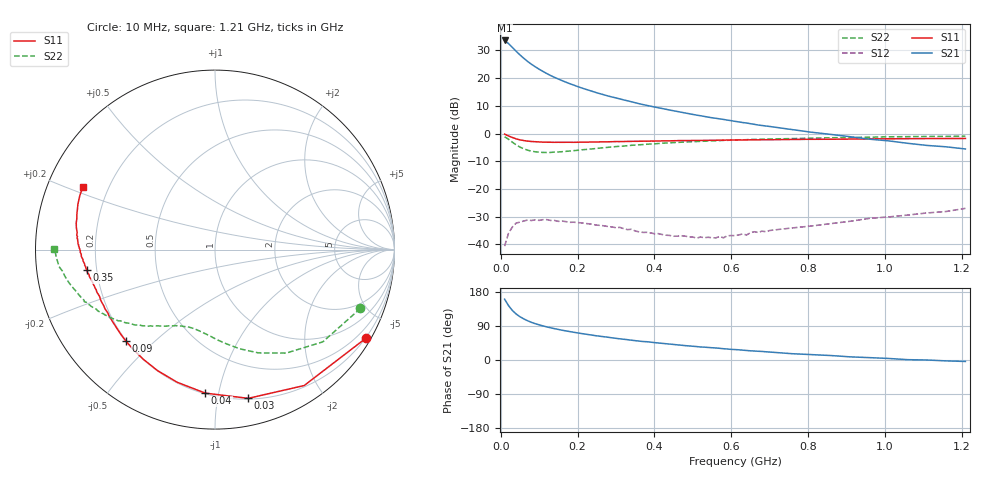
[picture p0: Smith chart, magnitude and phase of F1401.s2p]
! Fri Mar 13 15:56:18 1998
# MHZ  S  MA  R  50.0000
! SCATTERING PARAMETERS :
!  POLYFET RF DEVICES
!  F1401
!  S PARAMETERS
!  VDS=50V, IDQ=200mA
!FREQ  S11MAG S11ANG S21MAG S21ANG S12MAG S12ANG S22MAG S22ANG
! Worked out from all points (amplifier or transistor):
!   81 points, 10 MHz to 1.21 GHz, reference 50 ohm
!   highest |S21| = 33.6 dB at 10 MHz (marker M1)
!   |S21| within 3 dB of that: start of sweep to 33.68 MHz
!   unconditionally stable (mu >= 1): 227.7 MHz to end of sweep
!   at 140 MHz: K = 0.56, MSG = 25.8 dB, |S12| = -31.4 dB
!   at 410 MHz: K = 2.40, MAG = 16.1 dB, |S12| = -36.1 dB
!   at 1.21 GHz: K = 1.57, MAG = 6.3 dB, |S12| = -27.0 dB
!   S11 on the Smith chart (normalised r, x): 10 MHz: 0.18, -3.67; 30 MHz: 0.21, -1.23; 40 MHz: 0.20, -0.91; 90 MHz: 0.20, -0.41; 350 MHz: 0.16, -0.08; 1.21 GHz: 0.11, +0.22
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10  0.9751 -30.4  47.77 160.5  0.00929 68.9  0.8742 -22.0
20  0.9058 -56.7  42.06 143.8  0.01576 54.1  0.7906 -40.6
30  0.8491 -77.4  35.91 131.0  0.02051 45.1  0.7 -55.5
40  0.8014 -93.9  30.5 121.5  0.02424 36.0  0.6243 -67.2
50  0.7687 -105.9  26.21 114.2  0.02524 26.9  0.5698 -76.0
60  0.7465 -115.4  22.76 108.4  0.02641 23.7  0.5288 -83.1
70  0.7302 -123.2  19.96 103.5  0.02751 21.1  0.5012 -89.0
80  0.7186 -129.4  17.76 99.3  0.02696 16.1  0.4802 -93.8
90  0.7121 -134.2  15.98 95.8  0.02771 14.7  0.4682 -98.0
110  0.7001 -141.9  13.18 90.0  0.02794 9.8  0.4559 -104.5
130  0.6969 -147.5  11.11 84.9  0.02701 6.2  0.4566 -109.7
140  0.6936 -149.7  10.32 82.7  0.02706 4.5  0.4622 -111.9
170  0.696 -155.1  8.425 76.7  0.02574 1.9  0.4772 -117.4
210  0.6997 -160.2  6.668 69.8  0.02448 -0.6  0.5088 -123.0
280  0.709 -166.5  4.741 59.9  0.02093 -1.0  0.5647 -131.0
350  0.7244 -171.0  3.599 51.1  0.01749 1.0  0.619 -137.7
410  0.7337 -174.3  2.922 45.0  0.01565 9.8  0.66 -143.0
500  0.7492 -178.5  2.212 36.3  0.0136 27.7  0.713 -149.3
610  0.7649 176.9  1.66 27.5  0.01439 53.0  0.7627 -156.1
810  0.7874 169.1  1.054 14.2  0.02151 71.0  0.826 -165.9
1010  0.804 162.0  0.7376 4.1  0.03133 81.0  0.8736 -173.8
1210  0.815 154.7  0.5268 -3.8  0.0447 80.7  0.8959 180.0
